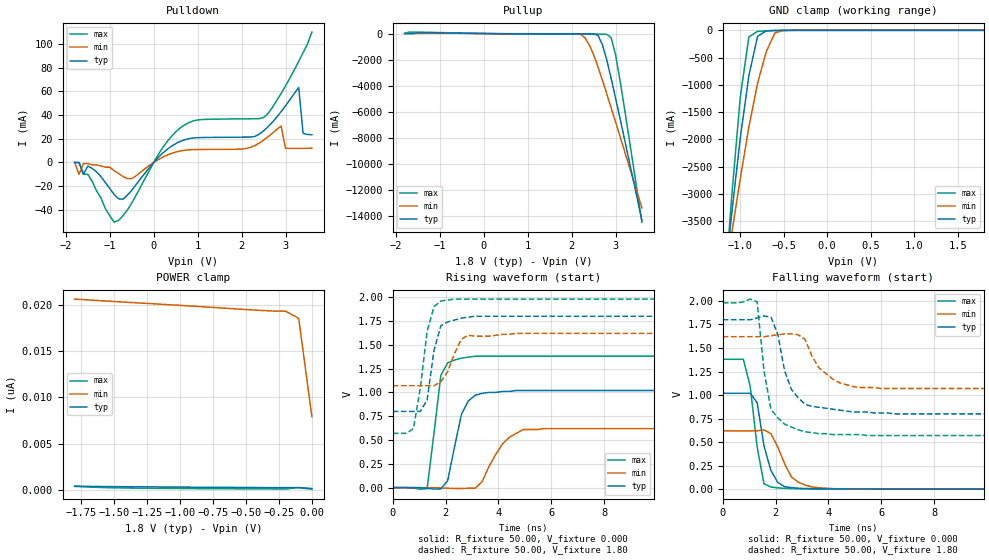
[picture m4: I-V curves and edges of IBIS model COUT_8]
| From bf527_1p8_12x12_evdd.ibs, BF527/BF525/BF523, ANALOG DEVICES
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|   Model prw0408swcdg_25
[Model]   COUT_8
Model_type   I/O
Polarity   Non-Inverting
Enable   Active-Low
Vinl =   0.70V
Vinh =   1.00V
Vmeas =   1.20V
Cref =  50.00pF
Rref =   1.00M
Vref =  0.000V
C_comp   4.57pF   4.11pF   5.03pF
[Temperature Range]   25.00   0.12k   -40.00
[Voltage Range]   1.80V   1.62V   1.98V
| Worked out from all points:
|   slope of the pulldown table from 0 to 0.27 V, typ, clamps not added: 27.1 ohm
|   slope of the pullup table from 0 to 0.27 V, typ, clamps not added: 26.9 ohm
|   GND clamp passes 1 mA (typ) near -0.53 V on its own axis
|   rising waveform, R_fixture 50.00, V_fixture 0.000: 20-80 % time 510ps typ, 811ps min, 359ps max; typ from 0 V to 1.02 V
|   rising waveform, R_fixture 50.00, V_fixture 1.80: 20-80 % time 380ps typ, 528ps min, 434ps max; typ from 0.8 V to 1.8 V
|   falling waveform, R_fixture 50.00, V_fixture 0.000: 20-80 % time 457ps typ, 633ps min, 388ps max; typ from 1.02 V to 0 V
|   falling waveform, R_fixture 50.00, V_fixture 1.80: 20-80 % time 660ps typ, 881ps min, 415ps max; typ from 1.8 V to 0.8 V
[Pulldown]
| voltage   I(typ)   I(min)   I(max)
-1.8V     0A         0A         0A
-1.7V     0A         -10mA      0A
-1.6V     -10mA      -1mA       -10mA
-1.4V     -5mA       -2mA       -16mA
-800mV    -30.7mA    -9.3mA     -48.85mA
500mV     15.88mA    8.74mA     25.76mA
2.5V      26.66mA    18.81mA    37.95mA
2.9V      42.92mA    30.63mA    58.28mA
3V        47.86mA    11.94mA    64.57mA
3.3V      63.22mA    11.88mA    85.31mA
3.4V      24.55mA    11.91mA    92.64mA
3.6V      23.36mA    12mA       110mA
[Pullup]
| voltage   I(typ)   I(min)   I(max)
-1.8V     1.53mA     550uA      10.64mA
-1.6V     3.01mA     560uA      110mA
2.2V      -22.71mA   -39.8mA    -37.75mA
2.3V      -23.18mA   -310mA     -37.82mA
2.4V      -25.42mA   -850mA     -37.94mA
2.6V      -130mA     -2.54A     -42.67mA
2.7V      -850mA     -3.56A     -49.74mA
2.8V      -2.01A     -4.61A     -61.07mA
2.9V      -3.43A     -5.68A     -310mA
3V        -4.93A     -6.76A     -1.61A
3.1V      -6.46A     -7.85A     -3.55A
3.6V      -14.31A    -13.35A    -14.44A
[GND_clamp]
| voltage   I(typ)   I(min)   I(max)
-1.8V     -14.28A    -11.35A    -18.41A
-1.2V     -4.9A      -4.81A     -5.19A
-1.1V     -3.4A      -3.75A     -3.1A
-1V       -1.99A     -2.73A     -1.24A
-900mV    -830mA     -1.77A     -120mA
-800mV    -110mA     -970mA     -19.21mA
-700mV    -9.89mA    -390mA     -9.78mA
-600mV    -2.57mA    -42.87mA   -3.5mA
-500mV    -460uA     -4.38mA    -550uA
1.8V      170pA      19.28nA    82.46pA
[POWER_clamp]
| voltage   I(typ)   I(min)   I(max)
-1.8V     420pA      20.63nA    400pA
-1.5V     370pA      20.37nA    240pA
-1.3V     350pA      20.2nA     200pA
-400mV    270pA      19.41nA    130pA
-200mV    260pA      19.32nA    110pA
-100mV    260pA      18.55nA    270pA
0V        170pA      7.92nA     95.65pA
[Ramp]
| variable   typ   min   max
dV/dt_r   0.61/0.47n   0.37/0.71n   0.83/0.28n
dV/dt_f   0.60/0.67n   0.33/0.77n   0.84/0.40n
R_load = 50.00
[Rising Waveform]
R_fixture = 50.00
V_fixture = 0.000
V_fixture_min = 0.000
V_fixture_max = 0.000
L_fixture = 0.000H
C_fixture = 0.000F
| time   V(typ)   V(min)   V(max)
0s        0V         0V         0V
1.3ns     -7.21mV    43.96uV    -11.21mV
1.82ns    -13.55mV   -3.1mV     1.18V
2.08ns    73.46mV    -6.38mV    1.31V
2.34ns    430mV      -9.69mV    1.34V
2.86ns    910mV      -6.49mV    1.37V
3.38ns    990mV      61.29mV    1.38V
4.16ns    1.01V      460mV      1.38V
4.94ns    1.02V      610mV      1.38V
13ns      1.02V      620mV      1.38V
[Rising Waveform]
R_fixture = 50.00
V_fixture = 1.80
V_fixture_min = 1.62
V_fixture_max = 1.98
L_fixture = 0.000H
C_fixture = 0.000F
| time   V(typ)   V(min)   V(max)
0s        800mV      1.07V      570mV
780ps     800mV      1.07V      620mV
1.04ns    800mV      1.07V      1.04V
1.3ns     920mV      1.07V      1.64V
1.56ns    1.44V      1.07V      1.9V
1.82ns    1.7V       1.11V      1.96V
2.08ns    1.74V      1.22V      1.97V
2.6ns     1.78V      1.56V      1.98V
2.86ns    1.79V      1.6V       1.98V
13ns      1.8V       1.62V      1.98V
[Falling Waveform]
R_fixture = 50.00
V_fixture = 0.000
V_fixture_min = 0.000
V_fixture_max = 0.000
L_fixture = 0.000H
C_fixture = 0.000F
| time   V(typ)   V(min)   V(max)
0s        1.02V      620mV      1.38V
780ps     1.02V      620mV      1.38V
1.04ns    1.02V      620mV      1.09V
1.3ns     920mV      620mV      450mV
1.56ns    460mV      630mV      57.18mV
1.82ns    200mV      590mV      23mV
2.08ns    72.42mV    450mV      13.38mV
2.6ns     16.17mV    130mV      6.68mV
3.38ns    5.63mV     23.43mV    2.15mV
13ns      -24.55uV   21.72uV    -33.69uV
[Falling Waveform]
R_fixture = 50.00
V_fixture = 1.80
V_fixture_min = 1.62
V_fixture_max = 1.98
L_fixture = 0.000H
C_fixture = 0.000F
| time   V(typ)   V(min)   V(max)
0s        1.8V       1.62V      1.98V
1.3ns     1.82V      1.62V      1.99V
1.56ns    1.84V      1.62V      1.26V
1.82ns    1.83V      1.63V      850mV
2.08ns    1.65V      1.64V      760mV
2.34ns    1.26V      1.65V      690mV
2.86ns    970mV      1.64V      630mV
3.64ns    870mV      1.29V      590mV
4.94ns    820mV      1.09V      580mV
13ns      800mV      1.07V      570mV
